(* Logix 5000 Rung export; software revision 16.04 *)

MODULES
   Local : vendor None type None code None
   MVI69E_AFC : vendor None type None code None
END_MODULES

TYPE AFCESiteAlarms :   // Indicates if a meter has any alarms
STRUCT
   Meter1 : BOOL;   // Meter in alarm
   Meter2 : BOOL;   // Meter in alarm
   Meter3 : BOOL;   // Meter in alarm
   Meter4 : BOOL;   // Meter in alarm
   Meter5 : BOOL;   // Meter in alarm
   Meter6 : BOOL;   // Meter in alarm
   Meter7 : BOOL;   // Meter in alarm
   Meter8 : BOOL;   // Meter in alarm
   Meter9 : BOOL;   // Meter in alarm
   Meter10 : BOOL;   // Meter in alarm
   Meter11 : BOOL;   // Meter in alarm
   Meter12 : BOOL;   // Meter in alarm
   Meter13 : BOOL;   // Meter in alarm
   Meter14 : BOOL;   // Meter in alarm
   Meter15 : BOOL;   // Meter in alarm
   Meter16 : BOOL;   // Meter in alarm
END_STRUCT
END_TYPE

TYPE AFCEFlag :   // Flags contains status information updated by ladder and also trigger bits for clock update
STRUCT
   AFCStopped : BOOL;   // Indicates that the module has sent a new input block to be processed by ladder - UPDATED BY LADDER
   AFCInputSequenceNum : INT;   // Meter number (0 -15) associated to blocks 1-16. Used to update "Profile" (meter type and product group.) UPDATED BY LADDER
END_STRUCT
END_TYPE

TYPE AFCEUtilBlockNonInterrupt :
STRUCT
   Now : BOOL;
   ModbusMasterCommand : BOOL;
   ModbusMasterResponse : BOOL;
   Archive : DINT;
   Prover : BOOL;
   PassThru : BOOL;
   Calibration : BOOL;
END_STRUCT
END_TYPE

TYPE AFCEMeterCalRequestActionType :
STRUCT
   ZeroShift : BOOL;   // Zero Shift
   SetZero : BOOL;   // Set Zero
   SetSpan : BOOL;   // Set Span
   SetMid1 : BOOL;   // Set Mid 1
   SetMid2 : BOOL;   // Set Mid 2
   SetMid3 : BOOL;   // Set Mid 3
END_STRUCT
END_TYPE

TYPE AFCEMeterLinearGas :   // Linear Gas Meter
STRUCT
   Control : AFCEMeterControl;   // Meter Control
   Status : AFCEMeterStatus;   // Meter Status
   ProcessVariables : AFCEMeterLinearGasProcess;   // Input process variables to be transferred to the module
   Analysis : AFCEMeterAnalysis;   // Molar Analysis data to be transferred to the module (only for gas products with online gas chromatograph applications)
   Alarm : AFCEMeterLinearGasAlarm;   // Meter Alarms
   Archive : AFCEMeterLinearGasArchive;   // Archive
   Profile : AFCEMeterProfile;   // Module profile (meter type/product group) transfered from the module
   Calibration : AFCEMeterLinearGasCal;   // Calibration
   BackPlaneReturn : AFCEMeterLinearGasBackPlaneReturn;
END_STRUCT
END_TYPE

TYPE AFCEProveConfigEnable :   // Prove controls at enable
STRUCT
   MeterNumber : INT;   // Meter number requested (1-16)
   AutoAcceptProve : BOOL;   // Auto-accept the prove
   AutoContinueProve : BOOL;   // Auto-continue the prove
END_STRUCT
END_TYPE

TYPE AFCEModbusGateway :   // Modbus Gateway
STRUCT
   Command : AFCEModbusGatewayCommand[10];   // Modbus gateway commands - contains setup and modbus data
END_STRUCT
END_TYPE

TYPE AFCEMeterCalRequestActionValue :
STRUCT
   ZeroShift : AFCEMeterCalRequestValue;   // Zero Shift
   SetZero : AFCEMeterCalRequestValue;   // Set Zero
   SetSpan : AFCEMeterCalRequestValue;   // Set Span
   SetMid1 : AFCEMeterCalRequestValue;   // Set Mid 1
   SetMid2 : AFCEMeterCalRequestValue;   // Set Mid 2
   SetMid3 : AFCEMeterCalRequestValue;   // Set Mid 3
END_STRUCT
END_TYPE

TYPE AFCEMeterAnalysisError :
STRUCT
   StreamOutOfRange : BOOL;   // Requested Stream Number Out of Range
   StreamNotConfigured : BOOL;   // Requested Stream Not Configured
END_STRUCT
END_TYPE

TYPE AFCEMeterLinearGasArchiveWrite :   // Write Archive
STRUCT
   Daily : BOOL;   // Set to 1 to write daily archive
   Hourly : BOOL;   // Set to 1 to write hourly archive
END_STRUCT
END_TYPE

TYPE AFCEMeterCalRequestValue :
STRUCT
   Applied : REAL;   // Applied
   Measured : REAL;   // Measured
END_STRUCT
END_TYPE

TYPE AFCEModbusMasterDataType :   // Modbus master data type
STRUCT
   Bit : BOOL;   // bit type
   Word : BOOL;   // word type (16-bit)
   Long : BOOL;   // long integer (32-bit)
   LongRemote : BOOL;   // long integer (32-bit)
END_STRUCT
END_TYPE

TYPE AFCEUtil :   // Used for internal ladder logic usage. These values must not be changed by user application.
STRUCT
   Flags : AFCEFlag;   // Wallclock update commands
   CycleCounter : INT;   // Reflects current block ID calculated by ladder to be sent to the module
   Buffer : AFCEUtilBuffer;
   Block : AFCEUtilBlock;
END_STRUCT
END_TYPE

TYPE AFCEWallclock :
STRUCT
   GetAFCTime : BOOL;   // Get current AFC Time
   SetAFCTimeFromPLCTime : BOOL;   // Set AFC time from PLC time. Updates current AFC time
   EnableLocalDateTime : BOOL;   // Enable Local Date Time.
   AFCTime : AFCETime;   // Coordinated Universal Time. Updated by either getting or setting AFC time.
END_STRUCT
END_TYPE

TYPE AFCEProvePhaseBitmap :   // AFC prove phase bitmap
STRUCT
   NotSelected : BOOL;   // Not selected
   Active : BOOL;   // Active, not counting
   CountingPast1stSwitch : BOOL;   // Counting past 1st switch for Udir and forward leg for Bdir)
   Past2ndSwitchFwdLeg : BOOL;   // Past 2nd switch forward leg (bidirectional only)
   Past1stSwithRetLeg : BOOL;   // Past 1st switch return leg (bidirectional only)
   RunComplete : BOOL;   // Run complete. past 2nd switch.
END_STRUCT
END_TYPE

TYPE AFCEMeterLinearGasCalRequest :
STRUCT
   ProcessVariable : AFCEMeterLinearGasCalRequestProces;   // Process Variable
   ActionType : AFCEMeterCalRequestActionType;   // Action Type
   Value : AFCEMeterCalRequestActionValue;   // Value
   Count : DINT;   // Number of calibration requests
END_STRUCT
END_TYPE

TYPE AFCEProveInputConfig :   // Prove input block results - prover configuration
STRUCT
   Type : INT;   // Prover type
   Options : INT;   // Prover options
   RunsPerProveTotal : INT;   // Total runs per prove
   RunsPerProveSelected : INT;   // Selected runs per prove
   MaxRunsBeforeAbort : INT;   // Max total runs before abort
   ShortPassesPerRun : INT;   // Short passes per run if bidir = 2 , else 0
END_STRUCT
END_TYPE

TYPE AFCEMeterCalResponse :
STRUCT
   Trigger : BOOL;   // Send Error Code and Values to module to be recorded
   ErrorCode : SINT;   // Error Code to send. 0-4 allowed. 0=No error. 1-4=User defined.
   Value : AFCEMeterCalRequestValue;   // Value to Send
   Count : DINT;   // Number of calibration responses
END_STRUCT
END_TYPE

TYPE AFCEMeterLinearGasAlarmControl :   // Linear Gas Process Alarms
STRUCT
   PulseFrequency : AFCEMeterProcessAlarm;   // Pulse Frequency Alarms
   Temperature : AFCEMeterProcessAlarm;   // Temperature Alarms
   Pressure : AFCEMeterProcessAlarm;   // Pressure Alarms
   MeterPulses : AFCEMeterProcessAlarmFidelity;   // Meter Pulses Alarms
END_STRUCT
END_TYPE

TYPE AFCEMeterArchiveFetchError :
STRUCT
   ArchiveSelectionInvalid : BOOL;   // Archive File Selection Invalid
   AgeOutsideSize : BOOL;   // Age Outside Configured File Size
   ArchiveNeverWritten : BOOL;   // Age OK but Archive Record Never Written (new or reconfigured meter)
   Reserverd1 : BOOL;
   Reserverd2 : BOOL;
   Reserverd3 : BOOL;
   Reserverd4 : BOOL;
   Reserverd5 : BOOL;
   Reserverd6 : BOOL;
   Reserverd7 : BOOL;
   Reserverd8 : BOOL;
   Reserverd9 : BOOL;
   Reserverd10 : BOOL;
   Reserverd11 : BOOL;
   Reserverd12 : BOOL;
   Reserverd13 : BOOL;
END_STRUCT
END_TYPE

TYPE AFCEModbusGatewayCommand :   // Modbus Gateway Command
STRUCT
   Config : AFCEModbusGatewayConfig;   // Config data to be entered by the user.
   Trigger : BOOL;   // Trigger the Command, when cleared module has responded.
   Data : INT[200];   // Contains modbus data written to the module (write commands)
END_STRUCT
END_TYPE

TYPE AFCEProveConfigAccept :   // Prove controls at accept. If auto-accept is selected must be available at enable
STRUCT
   RequestedInterpolationPoint : INT;   // Requested interpolation point (0 nearest)
   ApplyMFChangeAllStreams : BOOL;   // Apply change in meter factor to all streams
   ApplyMFChangeCurve : BOOL;   // Apply change in meter factor to all curve points
   ApplyNewMF : BOOL;   // CApply new meter factor
END_STRUCT
END_TYPE

TYPE AFCEModbusMasterCommand :   // Modbus Master Command
STRUCT
   Config : AFCEModbusMasterConfig;   // Modbus Master Configuration
   ErrorCode : INT;   // Error Code associated to Modbus Master Command
   Pending : BOOL;   // Pending Modbus Master Command - waiting for Modbus Response
   ReturnedTransactionID : DINT;   // Changes to Config.TransactionID value when response has returned.
   Data : INT[100];   // Read or Write Data
END_STRUCT
END_TYPE

TYPE AFCEMeterStatusMeter :   // Meter Status
STRUCT
   Enabled : BOOL;   // Meter Enable Status, 1=enabled
   EnableAlarm : BOOL;   // If set either: 1. The meter is not configured. 2. The event log is full, the action was not performed.
END_STRUCT
END_TYPE

TYPE AFCEMeterControl :   // Enable/Disable Meter and Streams
STRUCT
   Meter : AFCEMeterControlMeter;   // Control the Meter
   Stream : AFCEMeterControlStream;   // Control the Meter Streams
   ResetAccumulators : AFCEMeterSignals;   // Resets for meter accumulators
END_STRUCT
END_TYPE

TYPE AFCEProveSequencing :   // AFC prove sequencing tag for phase selection and ball positioning
STRUCT
   Phase : AFCEProvePhaseBitmap;   // AFC phase sequencing
   BallPositionReady : BOOL;   // Ball position: Ready (Udir & Bdir only; fwd leg Bdir)
   BallPositionSealed : BOOL;   // Ball position: Sealed (Udir & Bdir only; fwd leg Bdir)
   BallPositionReadyBwdLeg : BOOL;   // Ball position: Ready bwd leg (Bdir only)
   BallPositionSealedBwdLeg : BOOL;   // Ball position: Sealed bwd leg (Bdir only)
END_STRUCT
END_TYPE

TYPE AFCEMeterLinearGasAlarm :
STRUCT
   Control : AFCEMeterLinearGasAlarmControl;   // Alarm Control
END_STRUCT
END_TYPE

TYPE AFCEUtilBlockInterrupt :
STRUCT
   Now : BOOL;
   ModbusGateway : DINT;
   EnableDisable : BOOL;
   Analysis : DINT;
END_STRUCT
END_TYPE

TYPE AFCEComponents :   // High precision gas component analysis (only supported version 2.07.000)
STRUCT
   C1 : REAL;   // Methane
   N2 : REAL;   // Nitrogen
   CO2 : REAL;   // Carbon Dioxide
   C2 : REAL;   // Ethane
   C3 : REAL;   // Propane
   H20 : REAL;   // Water
   H2S : REAL;   // Hydrogen Sulphide
   H2 : REAL;   // Hydrogen
   CO : REAL;   // Carbon Monoxide
   O2 : REAL;   // Oxygen
   IC4 : REAL;   // Iso-butane
   NC4 : REAL;   // Normal Butane
   IC5 : REAL;   // Iso-pentane
   NC5 : REAL;   // Normal-pentane
   C6 : REAL;   // Hexane
   C7 : REAL;   // Heptane
   C8 : REAL;   // Octane
   C9 : REAL;   // Nonane
   C10 : REAL;   // Decane
   He : REAL;   // Helium
   Ar : REAL;   // Argon
   NeoC5 : REAL;   // Not Used
   UxUser1 : REAL;   // Not Used
   UyUser2 : REAL;   // Not Used
   UxUser3 : REAL;   // Not Used
   UyUser4 : REAL;   // Not Used
   UxUser5 : REAL;   // Not Used
   UyUser6 : REAL;   // Not Used
   UxUser7 : REAL;   // Not Used
   UyUser8 : REAL;   // Not Used
   UxUser9 : REAL;   // Not Used
   UyUser10 : REAL;   // Not Used
END_STRUCT
END_TYPE

TYPE AFCEMeterStatus :   // Status
STRUCT
   Meter : AFCEMeterStatusMeter;   // Meter Status
   Stream : AFCEMeterStatusStream;   // Stream Status
END_STRUCT
END_TYPE

TYPE AFCEUtilBlock :
STRUCT
   ProcessInput : INT;
   InterruptPending : AFCEUtilBlockInterrupt;
   InterruptComplete : AFCEUtilBlockInterrupt;
   NonInterruptPending : AFCEUtilBlockNonInterrupt;
   NonInterruptComplete : AFCEUtilBlockNonInterrupt;
END_STRUCT
END_TYPE

TYPE AFCEModbusGatewayConfig :   // Modbus Ggateway Configuration
STRUCT
   Enable : BOOL;   // Set to 1 to enable modbus gateway command (0=disable)
   StartRegister : DINT;   // Start modbus address
   RegisterCount : INT;   // Word count (200 max)
   FunctionType : BOOL;   // 0 = read command, 1 = write command
   RegisterType : BOOL;   // 0 = holding register, 1 = input register
   SlaveType : BOOL;   // 0 = primary slave, 1 = virtual slave
END_STRUCT
END_TYPE

TYPE AFCEMeterControlMeter :   // Enable and Disable Meter
STRUCT
   Enable : BOOL;   // Enable the Meter
   Disable : BOOL;   // Disable the Meter
END_STRUCT
END_TYPE

TYPE AFCEMeterProfile :   // Meter configuration profile
STRUCT
   MeterType : BOOL;   // 0=Differential, 1=Linear
   ProductGroup : BOOL;   // 0=Gas, 1=Liquid
   PrimaryInput : BOOL;   // For differential, 0=Differential Pressure 1=Flow Rate. For Linear, 0=Pulse Count 1=Pulse Frequency
   AOIMismatch : BOOL;   // AOI Meter type does not match module for meter number
END_STRUCT
END_TYPE

TYPE AFCEModbusPassThru :   // AFC Modbus Pass-thru
STRUCT
   Enable : BOOL;   // Set to 1 to enable pass-thru functionality (requires AFC Manager setting)
   MessagePresent : BOOL;   // Message present in the response block
   GetMessage : BOOL;   // Get the pass-thru message. When the bit is cleared the message has been transferred to the PLC.
   FunctionBitWrite : BOOL;   // Function bit write
   OverflowError : BOOL;   // Overflow error flag
   ModbusAddress : INT;   // Destination modbus address
   RegisterCount : INT;   // Number of elements associated to command
   ReadDataWord : INT[125];   // Contains received data for word commands
   ReadDataBit : AFCEModbusPassThruBitData;   // Contains received data for bit commands
END_STRUCT
END_TYPE

TYPE AFCEUtilBuffer :   // Buffer
STRUCT
   Input : INT[248];   // Input buffer contains the complete block to be copied from the module
   Output : INT[247];   // Output buffer contains data the complete block to be copied to the module
   Process : INT[180];
   ArchiveDay : INT[98];
   ArchiveHour : INT[98];
   Prove : INT[26];
   Analysis : INT[198];
   MeterEnableDisable : INT[4];
   StreamEnable : INT[36];
   StreamDisable : INT[36];
   StreamSelect : INT[24];
   MeterSignals : INT[24];
   Calibration : INT[36];
END_STRUCT
END_TYPE

TYPE AFCEProveStatus :   // Status of the prove (returned from the module to the processor)
STRUCT
   ProveAccepted : BOOL;   // Prove was accepted
   MeterFactorApplied : BOOL;   // Meter factor was applied
   MFAppliedToCurve : BOOL;   // Meter factor was applied to all points in the curve
   MFAppliedToStreams : BOOL;   // Meter factor was applied to all streams
   ProveRejectedByCommand : BOOL;   // Prove was rejected by command
   ProveRejectedNoRuns : BOOL;   // Prove was rejected - empty prove (no runs)
   ProveRejectedDivideBy0 : BOOL;   // Prove was rejected - divide by 0
   ProveEnabled : BOOL;   // Prove is enabled
   ProvingRunInProgress : BOOL;   // Proving run is in progress
   ProveRejectedAbort : BOOL;   // Prove rejected: abort
   ProvePaused : BOOL;   // Prove is paused
   RunCancelled : BOOL;   // Run Is cancelled
   RunTimedOut : BOOL;   // Run timed out
END_STRUCT
END_TYPE

TYPE AFCEMeterStatusStreamAlarm :   // Stream Alarms
STRUCT
   StreamOutOfRange : BOOL;   // Requested Stream Number Out of Range
   StreamNotConfigured : BOOL;   // Requested Stream not Configured
   StreamNotEnabled : BOOL;   // Requested Stream not Enabled
   EventLogFull : BOOL;   // Event Log Full, Action not Performed
END_STRUCT
END_TYPE

TYPE AFCEMeterLinearGasCal :   // Processor Mediated Calibration
STRUCT
   Request : AFCEMeterLinearGasCalRequest;   // Calibration Request from module
   Response : AFCEMeterCalResponse;   // Processor Response
END_STRUCT
END_TYPE

TYPE AFCEMeterLinearGasProcess :   // Linear Gas Process Variables
STRUCT
   PulseFrequency : REAL;   // Pulse Frequency (Hz)
   Temperature : REAL;   // Temperature
   Pressure : REAL;   // Pressure
   MeterPulses : DINT;   // Pulse count
END_STRUCT
END_TYPE

TYPE AFCEProveConfig :   // Controls (configuration settings) associated to the prover
STRUCT
   Enable : AFCEProveConfigEnable;   // Controls at enable
   Accept : AFCEProveConfigAccept;   // Controls at accept
END_STRUCT
END_TYPE

TYPE AFCESiteStatus :   // Site status bits - contains general information about the module - not meter specific
STRUCT
   AFCActive : BOOL;   // AFC active
   ChecksumAlarms : BOOL;   // Checkum alarm active
   Reserved2 : BOOL;
   Reserved3 : BOOL;
   PLCHalted : BOOL;   // PLC in program mode or missing
   CfgChanged : BOOL;   // Configuration changed
   Powerup : BOOL;   // Module powered up
   ColdStart : BOOL;   // Module performed cold start (BBRAM initialized)
   ModbusMasterPending : BOOL;   // Modbus Master Poll Pending
   ModbusMasterComplete : BOOL;   // Modbus Master Poll Complete
   ModbusPassThruPending : BOOL;   // Modbus Pass-thru Input Pending
   CalibrationRequest : BOOL;   // Calibration request from module
   ProverEnabled : BOOL;   // Prover Enabled
   Reserved13 : BOOL;
   Reserved14 : BOOL;
   Reserved15 : BOOL;
END_STRUCT
END_TYPE

TYPE AFCEModbusMaster :   // Modbus Master. Port 3 must be configured as modbus master through AFC Manager to use this feature.
STRUCT
   Enable : BOOL;   // Enable the modbus master funcionality
   CommandIndex : INT;   // Selects which command index will be executed
   Command : AFCEModbusMasterCommand[10];   // Each command contains a specific modbus request to be sent out of the port
END_STRUCT
END_TYPE

TYPE AFCEProveProcess :   // Prove process output from processor to the module
STRUCT
   Sequencing : AFCEProveSequencing;   // Prover sequencing
   Temperature : REAL;   // Temperature for Single Probe provers. And Inlet Temperature for Dual Probe Provers.
   OutletTemperature : REAL;   // Outlet Temperature for Provers with Dual Probes.
   SwitchBarTemperature : REAL;   // Switch bar temperature
   Pressure : REAL;   // Pressure for Single Probe provers. And Inlet Pressure for Dual Probe Provers.
   OutletPressure : REAL;   // Outlet Pressure for Provers with Dual Probes.
   ProverDensity : REAL;   // Prover density
END_STRUCT
END_TYPE

TYPE AFCEExtended :
STRUCT
   Trigger : BOOL;
   Data : AFCEExtendedData;
END_STRUCT
END_TYPE

TYPE AFCEMeterSignals :   // Meter trigger accumulator and archive resets
STRUCT
   ResetAccumulator1 : BOOL;   // Set to 1 to reset resettable accumulator 1
   ResetAccumulator2 : BOOL;   // Set to 1 to reset resettable accumulator 2
   ResetAccumulator3 : BOOL;   // Set to 1 to reset resettable accumulator 3
   ResetAccumulator4 : BOOL;   // Set to 1 to reset resettable accumulator 4
END_STRUCT
END_TYPE

TYPE AFCEMeterProcessAlarm :   // Process Alarms
STRUCT
   SetGeneralFail : BOOL;   // Set to indicate General Failure of the Transmitter
   StaleData : BOOL;   // Clear to Indicate new process input data
   SetLowThreshold : BOOL;   // Set to indicate Lower Range Limit Exceeded
   SetHighThreshold : BOOL;   // Set to indicate Upper Range Limit Exceeded
   SetAutoClearStaleData : BOOL;   // Set to automatically clear stale data
END_STRUCT
END_TYPE

TYPE AFCEMeterLinearGasArchive :   // Linear Gas Archive
STRUCT
   Write : AFCEMeterLinearGasArchiveWrite;
   Fetch : AFCEMeterLinearGasArchiveFetch;
END_STRUCT
END_TYPE

TYPE AFCETime :   // AFC time format used for wallclock update.
STRUCT
   Year : DINT;   // Year
   Month : DINT;   // Month
   Day : DINT;   // Day
   Hour : DINT;   // Hour
   Minute : DINT;   // Minute
   second : DINT;   // Seconds
END_STRUCT
END_TYPE

TYPE AFCEModbusMasterSwap :   // Modbus master swap words/ swap bytes
STRUCT
   SwapWords : BOOL;   // Swap words
   SwapBytes : BOOL;   // Swap bytes
END_STRUCT
END_TYPE

TYPE AFCEMeterControlStream :
STRUCT
   Selected : SINT;   // Stream to Enable or Disable and/or make active.
   EnableSelected : BOOL;   // Enable the Selected Stream
   DisableSelected : BOOL;   // Disable the Selected Stream
   SetSelectedToActive : BOOL;   // Set Selected to Active Stream
END_STRUCT
END_TYPE

TYPE AFCEProvePulseCount :   // Values to be supplied at the end of the pass/run
STRUCT
   Meter : DINT;   // Meter pulse count
   MasterMeter : DINT;   // Master meter pulse count
END_STRUCT
END_TYPE

TYPE AFCEMeterStatusStream :
STRUCT
   Active : INT;   // Current Active Stream
   Enabled : AFCEMeterStatusStreamEnabled;   // Enabled Streams
   Configured : AFCEMeterStatusStreamEnabled;   // Configured Streams
   EnableAlarm : AFCEMeterStatusStreamAlarm;   // Enable Alarms
END_STRUCT
END_TYPE

TYPE AFCEExtendedData :
STRUCT
   Raw : INT[64];
END_STRUCT
END_TYPE

TYPE AFCEModbusPassThruBitData :   // AFC Modbus Pass-thru Bit Data
STRUCT
   Data : BOOL[2016];   // Contains received data for bit commands
END_STRUCT
END_TYPE

TYPE AFCEMeterLinearGasArchiveFetch :
STRUCT
   Daily : AFCEMeterLinearGasArchiveFetchT;
   Hourly : AFCEMeterLinearGasArchiveFetchT;
END_STRUCT
END_TYPE

TYPE AFCEModbusMasterConfig :   // Modbus master command settings
STRUCT
   Enable : BOOL;   // Set to 1 to enable command (0=disable)
   FunctionType : BOOL;   // Set to 1 to select write command (0=read command)
   RegisterBank : BOOL;   // Set to 1 to select input register (0=holding register)
   DataType : AFCEModbusMasterDataType;   // Select data type format
   SwapOption : AFCEModbusMasterSwap;   // Select byte and word swap (1 = swap, 0 = no swap)
   TypeSwap : INT;   // This value is calculated by ladder logic and must not be modified by user
   SlaveAddress : INT;   // Modbus slave address of remote device
   ModbusAddress : INT;   // Modbus data address on remote slave
   ElementCount : INT;   // Number of data elements (125 words)
   TransactionID : INT;   // Transaction ID. This value is returned to the ReturnedTransaction ID when the response has been received.
END_STRUCT
END_TYPE

TYPE AFCEMeterProcessAlarmFidelity :   // Process Alarms
STRUCT
   SetGeneralFail : BOOL;   // Set to indicate General Failure of the Transmitter
   StaleData : BOOL;   // Clear to Indicate new process input data
   Reserved : BOOL;   // Reserved
   SetPulseFidelityAlarm : BOOL;   // Set to indicate Pulse Fidelity Alarm
   SetAutoClearStaleData : BOOL;   // Set to automatically clear stale data
END_STRUCT
END_TYPE

TYPE AFCEMeterLinearGasStandardDataDflt :   // EAFC Backplane Return Standard Data
STRUCT
   Meter_Alarms : DINT;   // Meter alarms
   NR_Acc_Net_Totalizer : DINT;   // Non-resettable accumulator, net, totalizer (m3)
   NR_Acc_Net_Residue : REAL;   // Non-resettable accumulator, net, residue (m3)
   FlowRate_Net : REAL;   // Flow rate, net (m3/h)
   FlowRate_Gross : REAL;   // Flow rate, gross / indicated (m3/h)
   Ifpv : REAL;   // AGA 8, Supercompressibility, Fpv
   Cprime : REAL;   // C-prime
END_STRUCT
END_TYPE

TYPE AFCEMeterLinearGasBackPlaneReturn :   // Linear Gas Meter
STRUCT
   StandardDefault : AFCEMeterLinearGasStandardDataDflt;
   StandardRaw : INT[14];
   Extended : AFCEExtended;
END_STRUCT
END_TYPE

TYPE AFCEMeterLinearGasCalRequestProces :
STRUCT
   PulseFrequency : BOOL;   // Pulse Frequency
   Temperature : BOOL;   // Temperature
   Pressure : BOOL;   // Pressure
END_STRUCT
END_TYPE

TYPE AFCEMeterLinearGasArchiveDflt :   // Default Configuration
STRUCT
   ClosingTimestamp : DINT;
   CumulativeActiveStreams : INT;
   CurrentActiveStream : SINT;
   MeterStatus : SINT;
   FlowingPeriod : DINT;
   PeriodDuration : DINT;
   AccumulatorTotalizer : DINT;
   AccumulatorResidue : REAL;
   MeterAlarms : DINT;
   PulseFrequency : REAL;
   Temperature : REAL;
   Pressure : REAL;
   RelativeDensity : REAL;
   ReferenceCompressibility : REAL;
   FlowingCompressibility : REAL;
   Fpv : REAL;
   KFactor : REAL;
   MeterFactor : REAL;
   InputPulseCount : DINT;
   CurrentManPulseCount : DINT;
   MassNRAccumulatorCurrent : REAL;   // Non-resettable
   MassNRAccumulatorOpening : REAL;   // Non-resettable
   EnergyNRAccumulatorCurrent : REAL;   // Non-resettable
   EnergyNRAccumulatorOpening : REAL;   // Non-resettable
   NetNRAccumulatorCurrent : REAL;   // Non-resettable
   NetNRAccumulatorOpening : REAL;   // Non-resettable
   GrossNRAccumulatorCurrent : REAL;   // Non-resettable
   GrossNRAccumulatorOpening : REAL;   // Non-resettable
   MolarFractionComponent01_C1 : REAL;
   MolarFractionComponent02_N2 : REAL;
   MolarFractionComponent03_CO2 : REAL;
   MolarFractionComponent04_C2 : REAL;
   MolarFractionComponent05_C3 : REAL;
   MolarFractionComponent06_H2O : REAL;
   MolarFractionComponent07_H2S : REAL;
   MolarFractionComponent08_H2 : REAL;
   MolarFractionComponent09_CO : REAL;
   MolarFractionComponent10_O2 : REAL;
   MolarFractionComponent11_IC4 : REAL;
   MolarFractionComponent12_NC4 : REAL;
   MolarFractionComponent13_IC5 : REAL;
   MolarFractionComponent14_NC5 : REAL;
   MolarFractionComponent15_C6 : REAL;
   MolarFractionComponent16_C7 : REAL;
   MolarFractionComponent17_C8 : REAL;
   MolarFractionComponent18_C9 : REAL;
   MolarFractionComponent19_C10 : REAL;
   MolarFractionComponent20_He : REAL;
   MolarFractionComponent21_Ar : REAL;
   UserSpecifiedFlowAverage1 : REAL;
   UserSpecifiedFlowAverage2 : REAL;
   UserSpecifiedFlowAverage3 : REAL;
END_STRUCT
END_TYPE

TYPE AFCEModuleDef :   // Main user defined data type
STRUCT
   ModbusGateway : AFCEModbusGateway;   // Reads and write data between processor and module modbus table
   ModbusMaster : AFCEModbusMaster;   // Setup modbus master commands to be sent to remote slaves (through Port 3)
   ModbusPassThru : AFCEModbusPassThru;   // Modbus pass-thru data
   SiteStatus : AFCESiteStatus;   // Site status
   MeterAlarms : AFCESiteAlarms;   // Meter Alarms
   Prove : AFCEProve;   // Prover
   Wallclock : AFCEWallclock;   // Set clock and get clock information
   Firmware : AFCEFirmwareVersion;   // Firmware information
   Util : AFCEUtil;   // Used by ladder logic
END_STRUCT
END_TYPE

TYPE AFCEMeterAnalysis :   // Meter analysis components. Allows the processor to update molar analysis for low precision and high precision streams.
STRUCT
   Trigger : BOOL;   // Set to 1 to Send Updated Component Data to the Module
   Stream : INT;   // Stream for Analysis. Select 0 for current active stream.
   Error : AFCEMeterAnalysisError;   // Analysis Error
   Components : AFCEComponents;   // High precision gas components (floating point per component). Only supported for firmware version 2.07.000 or later
END_STRUCT
END_TYPE

TYPE AFCEProveSignals :   // Contains the proving signals that will trigger specific tasks from the module
STRUCT
   EnableProve : BOOL;   // Enables the prove
   AcceptProve : BOOL;   // Accepts the prove
   RejectProve : BOOL;   // Reject the prove
   RunStart : BOOL;   // Starts the run
   RunComplete : BOOL;   // Flags that the run is complete
   RunCancel : BOOL;   // Cancels the run
   RunDelete : BOOL;   // Deletes the run
   PassComplete : BOOL;   // Flag that the pass is complete
   PauseProve : BOOL;   // Pauses the Proving Process
   AbortProve : BOOL;   // Aborts the prove
END_STRUCT
END_TYPE

TYPE AFCEFirmwareVersion :
STRUCT
   Major : SINT;   // Major Version number
   Minor : SINT;   // Minor Version number
   Revision : INT;   // Revision
END_STRUCT
END_TYPE

TYPE AFCEMeterLinearGasArchiveFetchT :   // Fetch Archive
STRUCT
   Trigger : BOOL;   // Trigger Archive Fetch
   Age : INT;   // 0 = Current Archive
   Error : AFCEMeterArchiveFetchError;   // Archive Fetch Error
   Default : AFCEMeterLinearGasArchiveDflt;   // Default Archive
   Raw : INT[100];   // Raw Archive
END_STRUCT
END_TYPE

TYPE AFCEProveRunResults :   // Run results of the prove. Copied from the module to the pocessor
STRUCT
   CountAttempted : INT;   // Run count attempted
   CountCompleted : INT;   // Run count completed
   CountSelected : INT;   // Run count selected
   RunsSelected : INT;   // Bit Mapped Runs selected for calculations from completed runs
   NewMeterFactor : REAL;   // New meter factor
   ChangeInMeterFactor : REAL;   // Change in meter factor
END_STRUCT
END_TYPE

TYPE AFCEMeterStatusStreamEnabled :   // Stream Status 1 = Enabled
STRUCT
   Stream1 : BOOL;
   Stream2 : BOOL;
   Stream3 : BOOL;
   Stream4 : BOOL;
   Stream5 : BOOL;
   Stream6 : BOOL;
   Stream7 : BOOL;
   Stream8 : BOOL;
   Stream9 : BOOL;
   Stream10 : BOOL;
   Stream11 : BOOL;
   Stream12 : BOOL;
   Stream13 : BOOL;
   Stream14 : BOOL;
   Stream15 : BOOL;
   Stream16 : BOOL;
END_STRUCT
END_TYPE

TYPE AFCEProve :   // Prove
STRUCT
   Process : AFCEProveProcess;   // Process Variables
   Signals : AFCEProveSignals;   // AFC Prove Signals (triggers the proving update)
   Config : AFCEProveConfig;   // AFC Prove Control (configuration settings)
   PulseCounts : AFCEProvePulseCount;   // Pulse counts to be updated at the end of the run/pass
   ConfigInput : AFCEProveInputConfig;   // AFC prover input configuration
   Status : AFCEProveStatus;   // AFC prover status
   ErrorCode : INT;   // Prove error code
   ProveControlsEcho : INT;   // AFC module Echos the state of the Prove Controls
   RequestedMeterEcho : INT;   // AFC module Echos the Meter number requested
   RequestedCurvePointEcho : INT;   // AFC module Echos the requested Curve Point
   RunResults : AFCEProveRunResults;   // Prove and run results
   ProveEnabled : BOOL;   // ON if prove is enabled. This flag is coped from inputbuffer[247]
END_STRUCT
END_TYPE

ADD_ON_INSTRUCTION AOI69EAFCMeterLinearGas   (* revision 1.5, vendor ProSoft Technology Inc., ExecutePrescan *)
// Add-On instruction for the MVI69E-AFC.
// Linear Gas Meter
// Revision note:
// Updated  BackplaneReturn Tag name from ProcessInputs to Standard
// and ComponentAnalysis to Extended.
// Help:
// Compatible with version 4.04 of MVI69E-AFC firmware or higher.
// v1.1: Comp Analysis Return fix
// v1.2: Addition of default process input backplane return data mapping.
// v1.3: Made correlation changes between the Module Archive Default UDTs and the AOI Archive Default UDTs.
// v1.4: Made changes to the Flow Rate Primary Input Block ID Insertion in Rung 8 (Removed +1),
// Modified ModbusGatewayConfig UDT StartRegister Tag Data Type from INT to DINT.
// v1.5: Updated Tags names AFCMeterXXYYYYYY.BackPlaneReturn.ProcessInputs to
// AFCMeterXXYYYYYY.BackPlaneReturn.Standard and
// AFCMeterXXYYYYYY.BackPlaneReturn.ComponentAnalysis
//  to AFCMeterXXYYYYYY.BackPlaneReturn.Extended.
VAR_IN_OUT
   ConnectionInput : INT[248]; {required}
   AFC : AFCEModuleDef; {required}
   AFCMeter : AFCEMeterLinearGas; {required}
END_VAR
VAR_INPUT
   MeterNumber : SINT; {required}   // Meter Number Set to a number between 1 and 12
END_VAR
VAR
   StreamSelectedShift : DINT;
   StreamSelectBuffer : INT;
   EnabledStatusBuffer : INT;
   StreamSelectBlockID : DINT;
   StreamNumberShift : DINT;
   StreamErrorBuffer : DINT;
   StreamEnableBlockID : DINT;
   StreamEnableBitPosition : DINT;
   StreamDisableBlockID : DINT;
   ProfileBuffer : SINT[2];
   ProcessInputBlockID : DINT;
   AnalysisGroupBitPosition : INT;
   AnalysisErrorBuffer : INT;
   ProcessAlarmShifter : DINT;
   ProcessAlarmBuffer : DINT;
   MeterSignaltBlockID : DINT;
   MeterNumberShift : DINT;
   MeterNumberBitPostition : DINT;
   Inputbuffer : INT[248];
   CalibrationMeterNumberBuffer : DINT;
   CalibrationMediationPending : BOOL;
   CalibrationInputScalingIndex : DINT;
   CalibrationHandleBuffer : DINT;
   ArchiveStream : DINT;
   ArchiveMeterStatusRaw : DINT;
   ArchiveMeterStatusActiveStream : DINT;
   ArchiveCompleteBitCheck : DINT;
   ArchiveBlockID : DINT;
   AnalysisGroupShift : DINT;
   AnalysisCompleteBitCheck : DINT;
   AnalysisBufferOffset : DINT;
   AnalysisBlockID : DINT;
   AFCStopped : BOOL;
   AFCInputDataAvailable : BOOL;
END_VAR

ROUTINE Logic   (* ladder *)
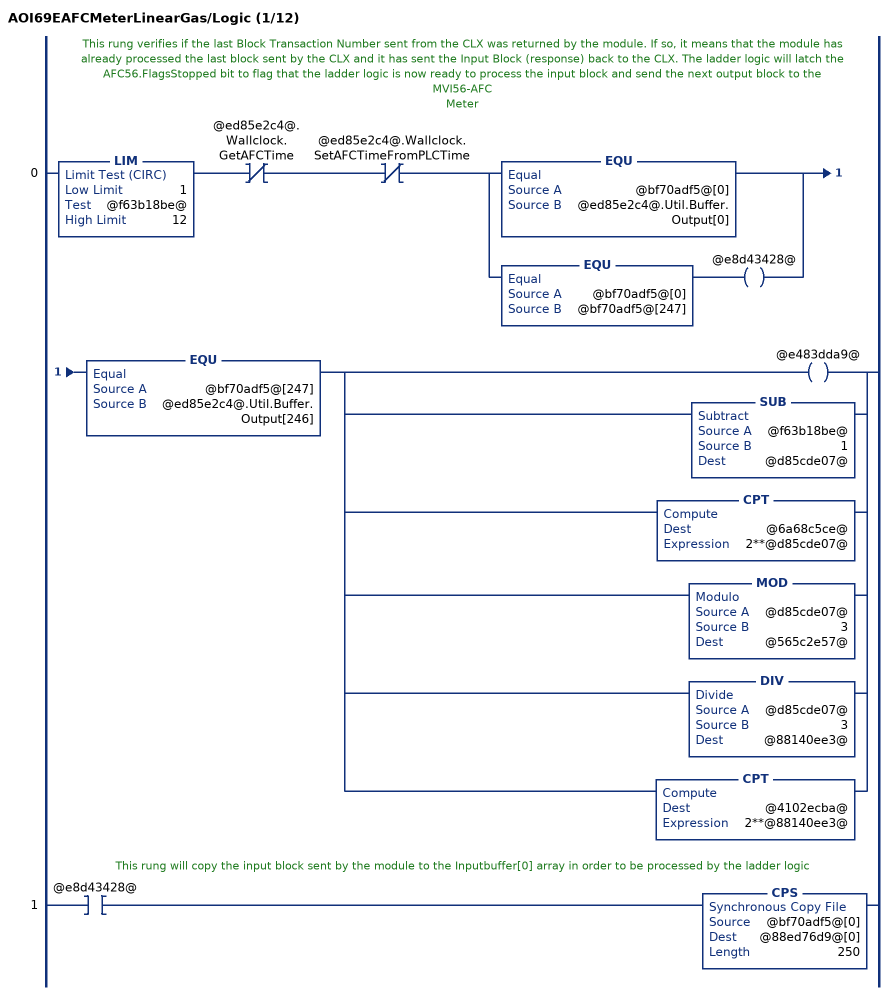
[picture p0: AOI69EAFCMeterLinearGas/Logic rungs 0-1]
   // This rung verifies if the last Block Transaction Number sent from the CLX was returned by the module. If so, it means that the module has already processed the last block sent by the CLX and it has sent the Input Block (response) back to the CLX. The ladder logic will latch the AFC56.FlagsStopped bit to flag that the ladder logic is now ready to process the input block and send the next output block to the MVI56-AFC
   // Meter
   0: LIM(1,@f63b18be@,12)XIO(@ed85e2c4@.Wallclock.GetAFCTime)XIO(@ed85e2c4@.Wallclock.SetAFCTimeFromPLCTime)[EQU(@bf70adf5@[0],@ed85e2c4@.Util.Buffer.Output[0]) ,EQU(@bf70adf5@[0],@bf70adf5@[247]) OTE(@e8d43428@) ]EQU(@bf70adf5@[247],@ed85e2c4@.Util.Buffer.Output[246])[OTE(@e483dda9@) ,SUB(@f63b18be@,1,@d85cde07@) ,CPT(@6a68c5ce@,2**@d85cde07@) ,MOD(@d85cde07@,3,@565c2e57@) ,DIV(@d85cde07@,3,@88140ee3@) ,CPT(@4102ecba@,2**@88140ee3@) ];
   // This rung will copy the input block sent by the module to the Inputbuffer[0] array in order to be processed by the ladder logic
   1: XIC(@e8d43428@)CPS(@bf70adf5@[0],@88ed76d9@[0],250);
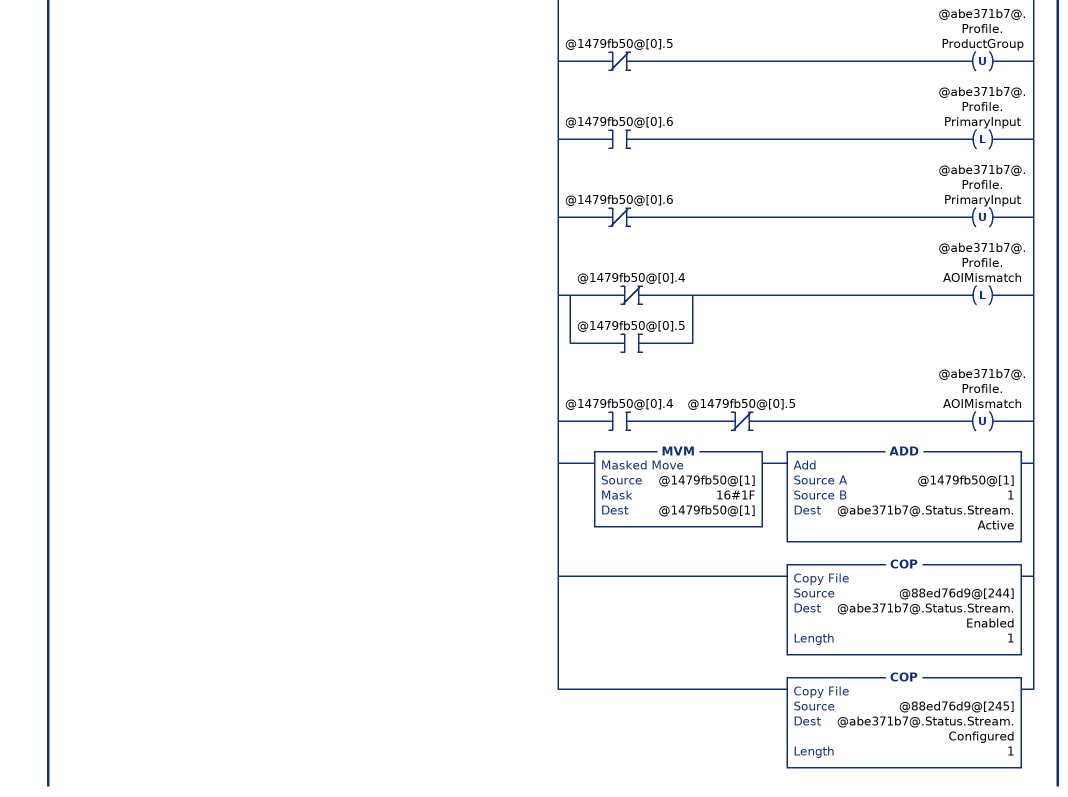
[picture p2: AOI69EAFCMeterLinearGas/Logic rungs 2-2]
   // Read process input backplane return and
   // meter profile (when block ID matches meter number).
   2: XIC(@e8d43428@)LIM(1,@88ed76d9@[0],12)[COP(@88ed76d9@[3+@d85cde07@*15],@abe371b7@.BackPlaneReturn.StandardRaw[0],14) ,COP(@abe371b7@.BackPlaneReturn.StandardRaw[0],@abe371b7@.BackPlaneReturn.StandardDefault,1) ,COP(@88ed76d9@[246],@ed85e2c4@.SiteStatus,1) ,EQU(@88ed76d9@[0],@f63b18be@) [COP(@88ed76d9@[243],@1479fb50@[0],2) ,[XIC(@1479fb50@[0].0) OTL(@abe371b7@.Status.Meter.EnableAlarm) ,XIO(@1479fb50@[0].0) OTU(@abe371b7@.Status.Meter.EnableAlarm) ] ,[XIC(@1479fb50@[0].1) OTL(@abe371b7@.Status.Meter.Enabled) ,XIO(@1479fb50@[0].1) OTU(@abe371b7@.Status.Meter.Enabled) ] ,[[XIC(@1479fb50@[0].4) OTL(@abe371b7@.Profile.MeterType) ,XIO(@1479fb50@[0].4) OTU(@abe371b7@.Profile.MeterType) ] ,[XIC(@1479fb50@[0].5) OTL(@abe371b7@.Profile.ProductGroup) ,XIO(@1479fb50@[0].5) OTU(@abe371b7@.Profile.ProductGroup) ] ,[XIC(@1479fb50@[0].6) OTL(@abe371b7@.Profile.PrimaryInput) ,XIO(@1479fb50@[0].6) OTU(@abe371b7@.Profile.PrimaryInput) ] ] ,[[XIO(@1479fb50@[0].4) ,XIC(@1479fb50@[0].5) ] OTL(@abe371b7@.Profile.AOIMismatch) ,XIC(@1479fb50@[0].4) XIO(@1479fb50@[0].5) OTU(@abe371b7@.Profile.AOIMismatch) ] ,MVM(@1479fb50@[1],16#1F,@1479fb50@[1]) ADD(@1479fb50@[1],1,@abe371b7@.Status.Stream.Active) ,COP(@88ed76d9@[244],@abe371b7@.Status.Stream.Enabled,1) ,COP(@88ed76d9@[245],@abe371b7@.Status.Stream.Configured,1) ] ];
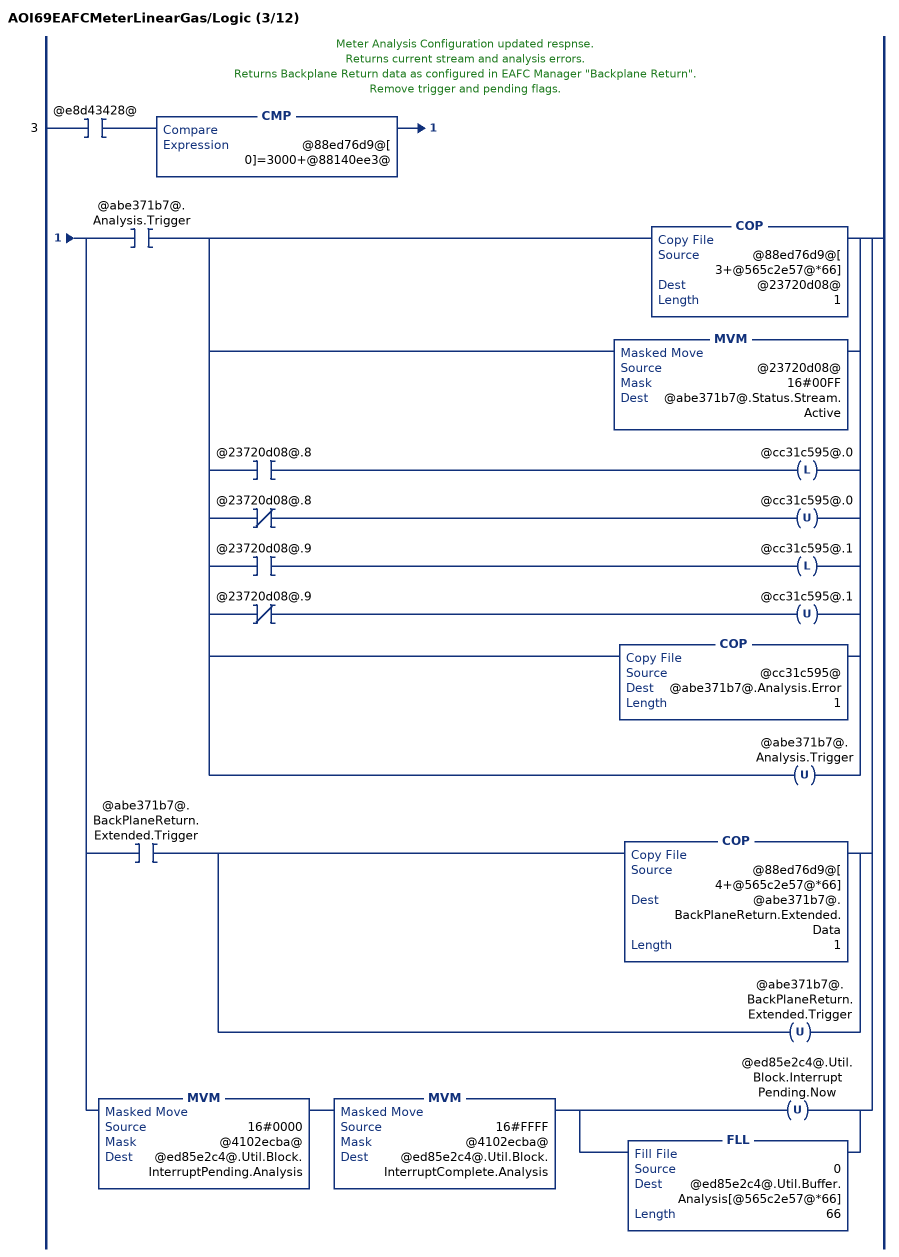
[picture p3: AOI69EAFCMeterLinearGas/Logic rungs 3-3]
   // Meter Analysis Configuration updated respnse.
   // Returns current stream and analysis errors.
   // Returns Backplane Return data as configured in EAFC Manager "Backplane Return".
   // Remove trigger and pending flags.
   3: XIC(@e8d43428@)CMP(@88ed76d9@[0]=3000+@88140ee3@)[XIC(@abe371b7@.Analysis.Trigger) [COP(@88ed76d9@[3+@565c2e57@*66],@23720d08@,1) ,MVM(@23720d08@,16#00FF,@abe371b7@.Status.Stream.Active) ,[XIC(@23720d08@.8) OTL(@cc31c595@.0) ,XIO(@23720d08@.8) OTU(@cc31c595@.0) ] ,[XIC(@23720d08@.9) OTL(@cc31c595@.1) ,XIO(@23720d08@.9) OTU(@cc31c595@.1) ] ,COP(@cc31c595@,@abe371b7@.Analysis.Error,1) ,OTU(@abe371b7@.Analysis.Trigger) ] ,XIC(@abe371b7@.BackPlaneReturn.Extended.Trigger) [COP(@88ed76d9@[4+@565c2e57@*66],@abe371b7@.BackPlaneReturn.Extended.Data,1) ,OTU(@abe371b7@.BackPlaneReturn.Extended.Trigger) ] ,MVM(16#0000,@4102ecba@,@ed85e2c4@.Util.Block.InterruptPending.Analysis) MVM(16#FFFF,@4102ecba@,@ed85e2c4@.Util.Block.InterruptComplete.Analysis) [OTU(@ed85e2c4@.Util.Block.InterruptPending.Now) ,FLL(0,@ed85e2c4@.Util.Buffer.Analysis[@565c2e57@*66],66) ] ];
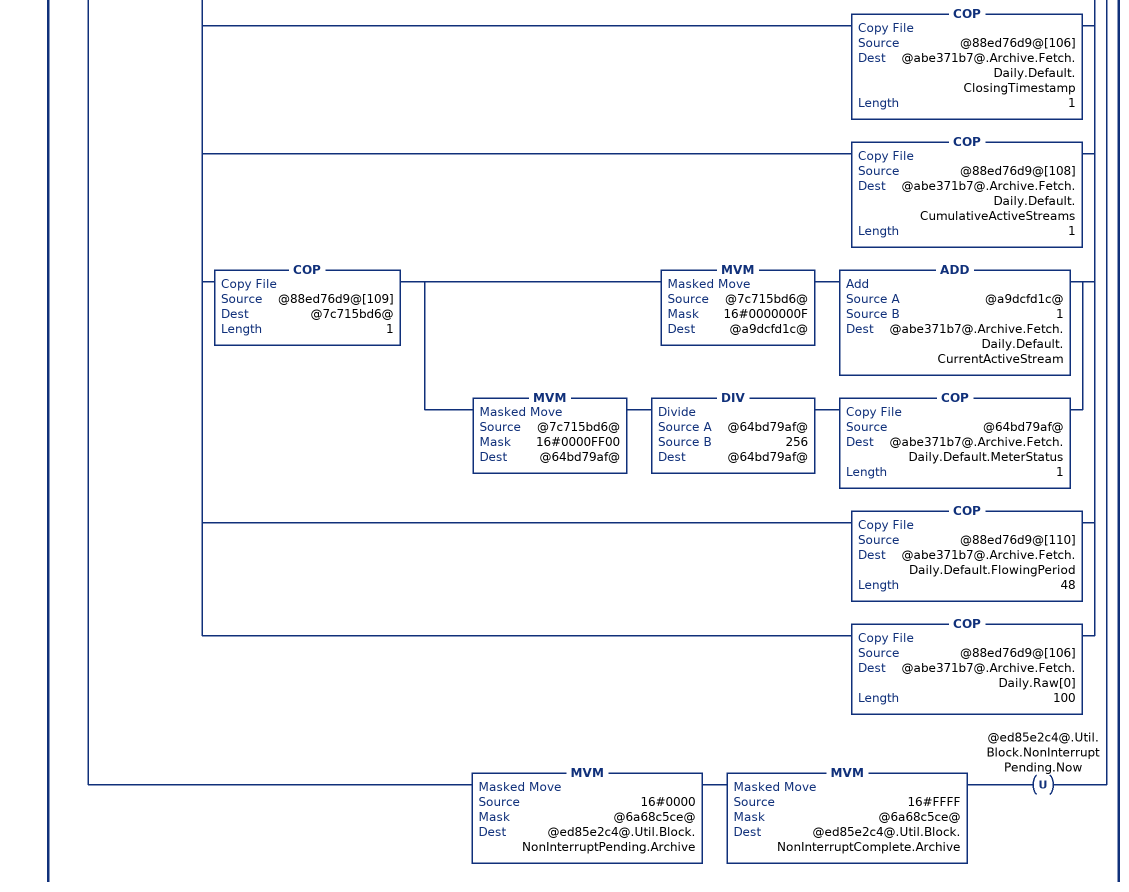
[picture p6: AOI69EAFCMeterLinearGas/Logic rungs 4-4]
   // Archive Fetch to default and raw UDT's.
   // Get archive alarms.
   // Remove trigger and pending flags.
   4: XIC(@e8d43428@)CMP(@88ed76d9@[0]=6000+@d85cde07@)[XIC(@abe371b7@.Archive.Fetch.Hourly.Trigger) [OTU(@abe371b7@.Archive.Fetch.Hourly.Trigger) ,[[XIC(@88ed76d9@[3].0) OTL(@abe371b7@.Archive.Fetch.Hourly.Error.ArchiveSelectionInvalid) ,XIO(@88ed76d9@[3].0) OTU(@abe371b7@.Archive.Fetch.Hourly.Error.ArchiveSelectionInvalid) ] ,[XIC(@88ed76d9@[3].1) OTL(@abe371b7@.Archive.Fetch.Hourly.Error.AgeOutsideSize) ,XIO(@88ed76d9@[3].1) OTU(@abe371b7@.Archive.Fetch.Hourly.Error.AgeOutsideSize) ] ,[XIC(@88ed76d9@[3].2) OTL(@abe371b7@.Archive.Fetch.Hourly.Error.ArchiveNeverWritten) ,XIO(@88ed76d9@[3].2) OTU(@abe371b7@.Archive.Fetch.Hourly.Error.ArchiveNeverWritten) ] ] ,COP(@88ed76d9@[4],@abe371b7@.Archive.Fetch.Hourly.Default.ClosingTimestamp,1) ,COP(@88ed76d9@[6],@abe371b7@.Archive.Fetch.Hourly.Default.CumulativeActiveStreams,1) ,COP(@88ed76d9@[7],@7c715bd6@,1) [MVM(@7c715bd6@,16#0000000F,@a9dcfd1c@) ADD(@a9dcfd1c@,1,@abe371b7@.Archive.Fetch.Hourly.Default.CurrentActiveStream) ,MVM(@7c715bd6@,16#0000FF00,@64bd79af@) DIV(@64bd79af@,256,@64bd79af@) COP(@64bd79af@,@abe371b7@.Archive.Fetch.Hourly.Default.MeterStatus,1) ] ,COP(@88ed76d9@[8],@abe371b7@.Archive.Fetch.Hourly.Default.FlowingPeriod,48) ,COP(@88ed76d9@[4],@abe371b7@.Archive.Fetch.Hourly.Raw[0],100) ] ,XIC(@abe371b7@.Archive.Fetch.Daily.Trigger) [OTU(@abe371b7@.Archive.Fetch.Daily.Trigger) ,[[XIC(@88ed76d9@[105].0) OTL(@abe371b7@.Archive.Fetch.Daily.Error.ArchiveSelectionInvalid) ,XIO(@88ed76d9@[105].0) OTU(@abe371b7@.Archive.Fetch.Daily.Error.ArchiveSelectionInvalid) ] ,[XIC(@88ed76d9@[105].1) OTL(@abe371b7@.Archive.Fetch.Daily.Error.AgeOutsideSize) ,XIO(@88ed76d9@[105].1) OTU(@abe371b7@.Archive.Fetch.Daily.Error.AgeOutsideSize) ] ,[XIC(@88ed76d9@[105].2) OTL(@abe371b7@.Archive.Fetch.Daily.Error.ArchiveNeverWritten) ,XIO(@88ed76d9@[105].2) OTU(@abe371b7@.Archive.Fetch.Daily.Error.ArchiveNeverWritten) ] ] ,COP(@88ed76d9@[106],@abe371b7@.Archive.Fetch.Daily.Default.ClosingTimestamp,1) ,COP(@88ed76d9@[108],@abe371b7@.Archive.Fetch.Daily.Default.CumulativeActiveStreams,1) ,COP(@88ed76d9@[109],@7c715bd6@,1) [MVM(@7c715bd6@,16#0000000F,@a9dcfd1c@) ADD(@a9dcfd1c@,1,@abe371b7@.Archive.Fetch.Daily.Default.CurrentActiveStream) ,MVM(@7c715bd6@,16#0000FF00,@64bd79af@) DIV(@64bd79af@,256,@64bd79af@) COP(@64bd79af@,@abe371b7@.Archive.Fetch.Daily.Default.MeterStatus,1) ] ,COP(@88ed76d9@[110],@abe371b7@.Archive.Fetch.Daily.Default.FlowingPeriod,48) ,COP(@88ed76d9@[106],@abe371b7@.Archive.Fetch.Daily.Raw[0],100) ] ,MVM(16#0000,@6a68c5ce@,@ed85e2c4@.Util.Block.NonInterruptPending.Archive) MVM(16#FFFF,@6a68c5ce@,@ed85e2c4@.Util.Block.NonInterruptComplete.Archive) OTU(@ed85e2c4@.Util.Block.NonInterruptPending.Now) ];
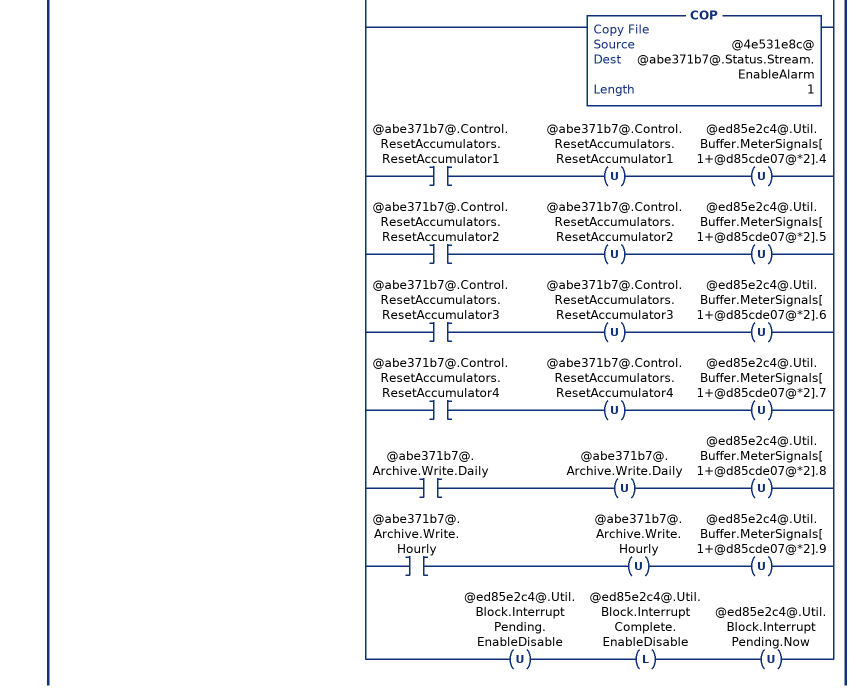
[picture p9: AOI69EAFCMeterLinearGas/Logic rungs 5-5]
   // Meter status and stream status.
   // Remove trigger and pending flags.
   5: XIC(@e8d43428@)EQU(@88ed76d9@[0],7000)[[MVM(@88ed76d9@[3],@6a68c5ce@,@da16ad6b@) ,[NEQ(@da16ad6b@,0) OTL(@abe371b7@.Status.Meter.Enabled) ,EQU(@da16ad6b@,0) OTU(@abe371b7@.Status.Meter.Enabled) ] ,OTU(@abe371b7@.Control.Meter.Enable) MVM(16#0000,@6a68c5ce@,@ed85e2c4@.Util.Buffer.MeterEnableDisable[1]) ,OTU(@abe371b7@.Control.Meter.Disable) MVM(16#0000,@6a68c5ce@,@ed85e2c4@.Util.Buffer.MeterEnableDisable[3]) ] ,[XIC(@abe371b7@.Control.Stream.EnableSelected) [COP(@88ed76d9@[7+@d85cde07@*3],@abe371b7@.Status.Stream.Enabled,1) ,COP(@88ed76d9@[8+@d85cde07@*3],@abe371b7@.Status.Stream.Configured,1) ,OTU(@abe371b7@.Control.Stream.EnableSelected) OTU(@abe371b7@.Control.Stream.DisableSelected) ] ,XIC(@abe371b7@.Control.Stream.DisableSelected) [COP(@88ed76d9@[55+@d85cde07@*3],@abe371b7@.Status.Stream.Enabled,1) ,COP(@88ed76d9@[56+@d85cde07@*3],@abe371b7@.Status.Stream.Configured,1) ,OTU(@abe371b7@.Control.Stream.EnableSelected) OTU(@abe371b7@.Control.Stream.DisableSelected) ] ] ,[OTU(@abe371b7@.Control.Stream.SetSelectedToActive) ,COP(@88ed76d9@[103+@d85cde07@*2],@23720d08@,1) ,[XIC(@23720d08@.8) OTL(@4e531e8c@.0) ,XIO(@23720d08@.8) OTU(@4e531e8c@.0) ] ,[XIC(@23720d08@.9) OTL(@4e531e8c@.1) ,XIO(@23720d08@.9) OTU(@4e531e8c@.1) ] ,[XIC(@23720d08@.10) OTL(@4e531e8c@.2) ,XIO(@23720d08@.10) OTU(@4e531e8c@.2) ] ,[XIC(@23720d08@.11) OTL(@4e531e8c@.3) ,XIO(@23720d08@.11) OTU(@4e531e8c@.3) ] ,MVM(@23720d08@,16#000F,@03251409@) ADD(@03251409@,1,@abe371b7@.Status.Stream.Active) ,COP(@4e531e8c@,@abe371b7@.Status.Stream.EnableAlarm,1) ] ,[XIC(@abe371b7@.Control.ResetAccumulators.ResetAccumulator1) OTU(@abe371b7@.Control.ResetAccumulators.ResetAccumulator1) OTU(@ed85e2c4@.Util.Buffer.MeterSignals[1+@d85cde07@*2].4) ,XIC(@abe371b7@.Control.ResetAccumulators.ResetAccumulator2) OTU(@abe371b7@.Control.ResetAccumulators.ResetAccumulator2) OTU(@ed85e2c4@.Util.Buffer.MeterSignals[1+@d85cde07@*2].5) ,XIC(@abe371b7@.Control.ResetAccumulators.ResetAccumulator3) OTU(@abe371b7@.Control.ResetAccumulators.ResetAccumulator3) OTU(@ed85e2c4@.Util.Buffer.MeterSignals[1+@d85cde07@*2].6) ,XIC(@abe371b7@.Control.ResetAccumulators.ResetAccumulator4) OTU(@abe371b7@.Control.ResetAccumulators.ResetAccumulator4) OTU(@ed85e2c4@.Util.Buffer.MeterSignals[1+@d85cde07@*2].7) ,XIC(@abe371b7@.Archive.Write.Daily) OTU(@abe371b7@.Archive.Write.Daily) OTU(@ed85e2c4@.Util.Buffer.MeterSignals[1+@d85cde07@*2].8) ,XIC(@abe371b7@.Archive.Write.Hourly) OTU(@abe371b7@.Archive.Write.Hourly) OTU(@ed85e2c4@.Util.Buffer.MeterSignals[1+@d85cde07@*2].9) ] ,OTU(@ed85e2c4@.Util.Block.InterruptPending.EnableDisable) OTL(@ed85e2c4@.Util.Block.InterruptComplete.EnableDisable) OTU(@ed85e2c4@.Util.Block.InterruptPending.Now) ];
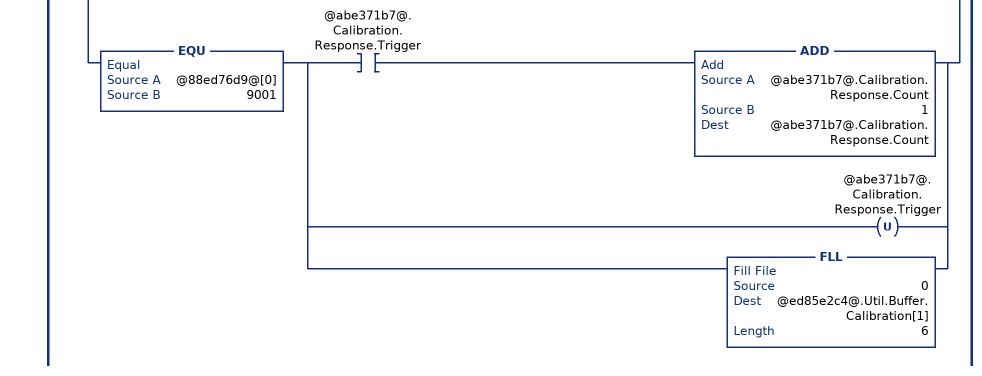
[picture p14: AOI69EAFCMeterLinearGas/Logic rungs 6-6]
   // Meter transmitter calibration.
   6: XIC(@e8d43428@)[EQU(@88ed76d9@[0],9000) ,EQU(@88ed76d9@[0],9001) ][MVM(@88ed76d9@[3],16#0F00,@624ee698@) ,DIV(@624ee698@,16#100,@624ee698@) ]EQU(@624ee698@,@d85cde07@)XIO(@88ed76d9@[3].14)[EQU(@88ed76d9@[0],9000) [XIO(@0ec75abb@) ADD(@abe371b7@.Calibration.Request.Count,1,@abe371b7@.Calibration.Request.Count) ,OTL(@0ec75abb@) [COP(@88ed76d9@[3],@6b8e262d@,1) ,MVM(@6b8e262d@,16#000F,@0e455032@) ] ,[EQU(@0e455032@,0) [OTL(@abe371b7@.Calibration.Request.ProcessVariable.PulseFrequency) ,OTU(@abe371b7@.Calibration.Request.ProcessVariable.Temperature) ,OTU(@abe371b7@.Calibration.Request.ProcessVariable.Pressure) ] ,EQU(@0e455032@,1) [OTL(@abe371b7@.Calibration.Request.ProcessVariable.Temperature) ,OTU(@abe371b7@.Calibration.Request.ProcessVariable.PulseFrequency) ,OTU(@abe371b7@.Calibration.Request.ProcessVariable.Pressure) ] ,EQU(@0e455032@,2) [OTL(@abe371b7@.Calibration.Request.ProcessVariable.Pressure) ,OTU(@abe371b7@.Calibration.Request.ProcessVariable.PulseFrequency) ,OTU(@abe371b7@.Calibration.Request.ProcessVariable.Temperature) ] ] ,[[XIC(@88ed76d9@[5].2) [OTL(@abe371b7@.Calibration.Request.ActionType.ZeroShift) ,COP(@88ed76d9@[6],@abe371b7@.Calibration.Request.Value.ZeroShift.Applied,2) ] ,XIO(@88ed76d9@[5].2) [OTU(@abe371b7@.Calibration.Request.ActionType.ZeroShift) ,FLL(0,@abe371b7@.Calibration.Request.Value.ZeroShift.Applied,2) ] ] ,[XIC(@88ed76d9@[5].3) [OTL(@abe371b7@.Calibration.Request.ActionType.SetZero) ,COP(@88ed76d9@[10],@abe371b7@.Calibration.Request.Value.SetZero.Applied,2) ] ,XIO(@88ed76d9@[5].3) [OTU(@abe371b7@.Calibration.Request.ActionType.SetZero) ,FLL(0,@abe371b7@.Calibration.Request.Value.SetZero.Applied,2) ] ] ,[XIC(@88ed76d9@[5].4) [OTL(@abe371b7@.Calibration.Request.ActionType.SetSpan) ,COP(@88ed76d9@[14],@abe371b7@.Calibration.Request.Value.SetSpan.Applied,2) ] ,XIO(@88ed76d9@[5].4) [OTU(@abe371b7@.Calibration.Request.ActionType.SetSpan) ,FLL(0,@abe371b7@.Calibration.Request.Value.SetSpan.Applied,2) ] ] ,[XIC(@88ed76d9@[5].5) [OTL(@abe371b7@.Calibration.Request.ActionType.SetMid1) ,COP(@88ed76d9@[18],@abe371b7@.Calibration.Request.Value.SetMid1.Applied,2) ] ,XIO(@88ed76d9@[5].5) [OTU(@abe371b7@.Calibration.Request.ActionType.SetMid1) ,FLL(0,@abe371b7@.Calibration.Request.Value.SetMid1.Applied,2) ] ] ,[XIC(@88ed76d9@[5].6) [OTL(@abe371b7@.Calibration.Request.ActionType.SetMid2) ,COP(@88ed76d9@[22],@abe371b7@.Calibration.Request.Value.SetMid2.Applied,2) ] ,XIO(@88ed76d9@[5].6) [OTU(@abe371b7@.Calibration.Request.ActionType.SetMid2) ,FLL(0,@abe371b7@.Calibration.Request.Value.SetMid2.Applied,2) ] ] ,[XIC(@88ed76d9@[5].7) [OTL(@abe371b7@.Calibration.Request.ActionType.SetMid3) ,COP(@88ed76d9@[26],@abe371b7@.Calibration.Request.Value.SetMid3.Applied,2) ] ,XIO(@88ed76d9@[5].7) [OTU(@abe371b7@.Calibration.Request.ActionType.SetMid3) ,FLL(0,@abe371b7@.Calibration.Request.Value.SetMid3.Applied,2) ] ] ] ] ,EQU(@88ed76d9@[0],9001) [XIC(@abe371b7@.Calibration.Response.Trigger) ADD(@abe371b7@.Calibration.Response.Count,1,@abe371b7@.Calibration.Response.Count) ,OTU(@abe371b7@.Calibration.Response.Trigger) ,FLL(0,@ed85e2c4@.Util.Buffer.Calibration[1],6) ] ];
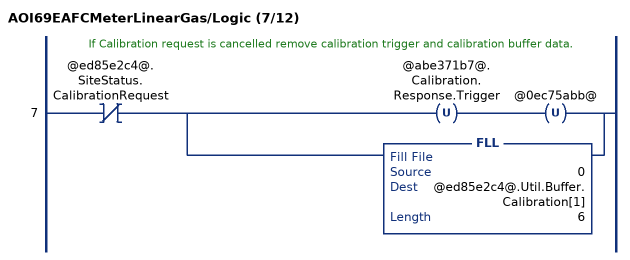
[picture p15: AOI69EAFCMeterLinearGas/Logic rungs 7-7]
   // If Calibration request is cancelled remove calibration trigger and calibration buffer data.
   7: XIO(@ed85e2c4@.SiteStatus.CalibrationRequest)[OTU(@abe371b7@.Calibration.Response.Trigger) OTU(@0ec75abb@) ,FLL(0,@ed85e2c4@.Util.Buffer.Calibration[1],6) ];
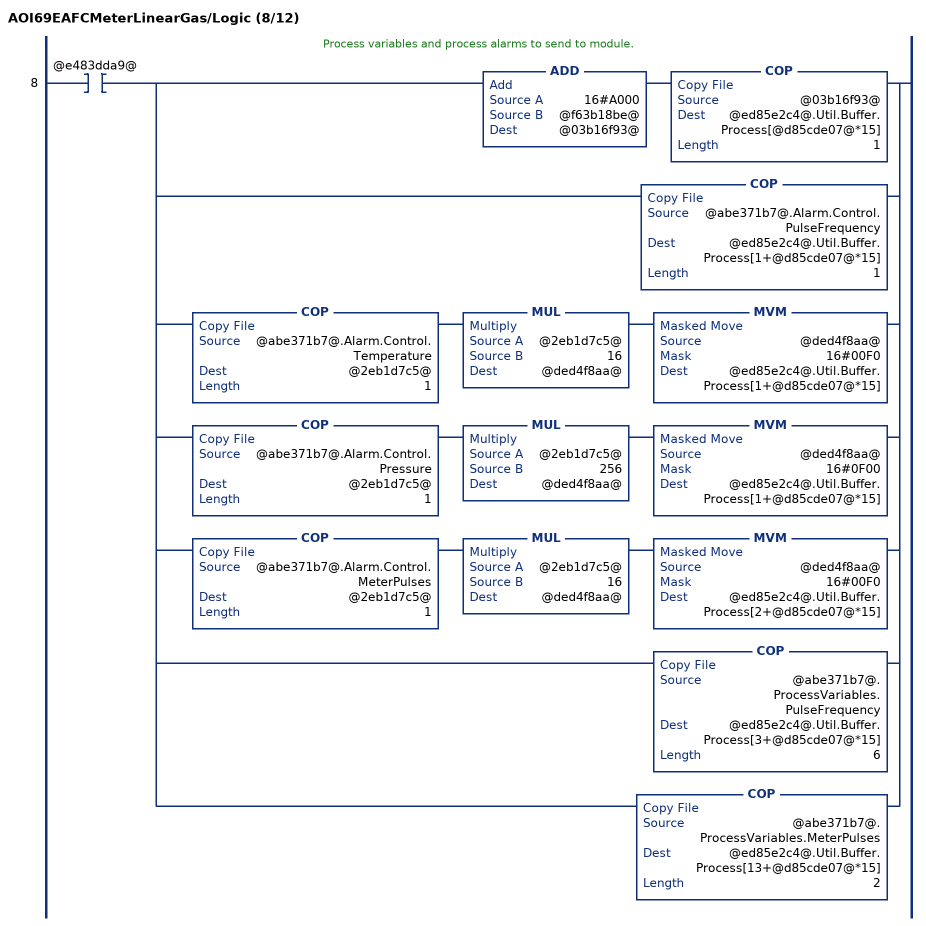
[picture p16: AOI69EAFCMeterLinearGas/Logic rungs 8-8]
   // Process variables and process alarms to send to module.
   8: XIC(@e483dda9@)[ADD(16#A000,@f63b18be@,@03b16f93@) COP(@03b16f93@,@ed85e2c4@.Util.Buffer.Process[@d85cde07@*15],1) ,COP(@abe371b7@.Alarm.Control.PulseFrequency,@ed85e2c4@.Util.Buffer.Process[1+@d85cde07@*15],1) ,COP(@abe371b7@.Alarm.Control.Temperature,@2eb1d7c5@,1) MUL(@2eb1d7c5@,16,@ded4f8aa@) MVM(@ded4f8aa@,16#00F0,@ed85e2c4@.Util.Buffer.Process[1+@d85cde07@*15]) ,COP(@abe371b7@.Alarm.Control.Pressure,@2eb1d7c5@,1) MUL(@2eb1d7c5@,256,@ded4f8aa@) MVM(@ded4f8aa@,16#0F00,@ed85e2c4@.Util.Buffer.Process[1+@d85cde07@*15]) ,COP(@abe371b7@.Alarm.Control.MeterPulses,@2eb1d7c5@,1) MUL(@2eb1d7c5@,16,@ded4f8aa@) MVM(@ded4f8aa@,16#00F0,@ed85e2c4@.Util.Buffer.Process[2+@d85cde07@*15]) ,[COP(@abe371b7@.ProcessVariables.PulseFrequency,@ed85e2c4@.Util.Buffer.Process[3+@d85cde07@*15],6) ,COP(@abe371b7@.ProcessVariables.MeterPulses,@ed85e2c4@.Util.Buffer.Process[13+@d85cde07@*15],2) ] ];
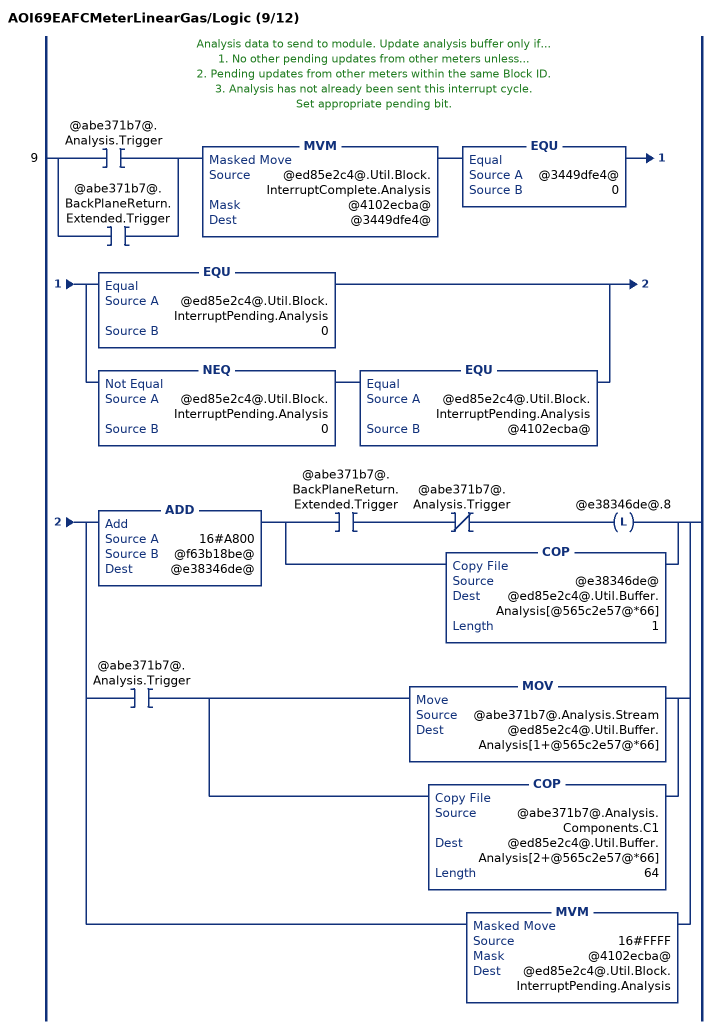
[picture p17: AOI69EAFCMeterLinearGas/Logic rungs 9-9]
   // Analysis data to send to module. Update analysis buffer only if...
   // 1. No other pending updates from other meters unless...
   // 2. Pending updates from other meters within the same Block ID.
   // 3. Analysis has not already been sent this interrupt cycle.
   // Set appropriate pending bit.
   9: [XIC(@abe371b7@.Analysis.Trigger) ,XIC(@abe371b7@.BackPlaneReturn.Extended.Trigger) ]MVM(@ed85e2c4@.Util.Block.InterruptComplete.Analysis,@4102ecba@,@3449dfe4@)EQU(@3449dfe4@,0)[EQU(@ed85e2c4@.Util.Block.InterruptPending.Analysis,0) ,NEQ(@ed85e2c4@.Util.Block.InterruptPending.Analysis,0) EQU(@ed85e2c4@.Util.Block.InterruptPending.Analysis,@4102ecba@) ][ADD(16#A800,@f63b18be@,@e38346de@) [XIC(@abe371b7@.BackPlaneReturn.Extended.Trigger) XIO(@abe371b7@.Analysis.Trigger) OTL(@e38346de@.8) ,COP(@e38346de@,@ed85e2c4@.Util.Buffer.Analysis[@565c2e57@*66],1) ] ,XIC(@abe371b7@.Analysis.Trigger) [MOV(@abe371b7@.Analysis.Stream,@ed85e2c4@.Util.Buffer.Analysis[1+@565c2e57@*66]) ,COP(@abe371b7@.Analysis.Components.C1,@ed85e2c4@.Util.Buffer.Analysis[2+@565c2e57@*66],64) ] ,MVM(16#FFFF,@4102ecba@,@ed85e2c4@.Util.Block.InterruptPending.Analysis) ];
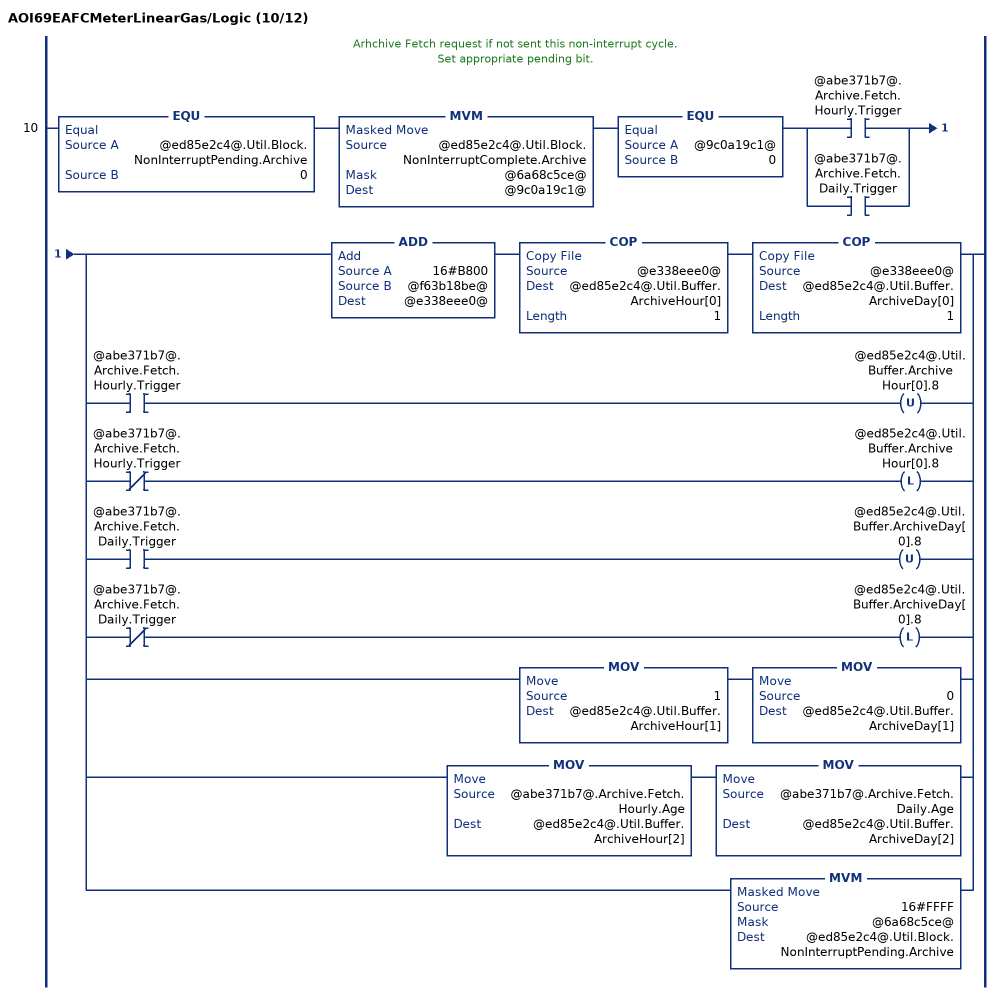
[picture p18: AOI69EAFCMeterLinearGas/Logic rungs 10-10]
   // Arhchive Fetch request if not sent this non-interrupt cycle.
   // Set appropriate pending bit.
   10: EQU(@ed85e2c4@.Util.Block.NonInterruptPending.Archive,0)MVM(@ed85e2c4@.Util.Block.NonInterruptComplete.Archive,@6a68c5ce@,@9c0a19c1@)EQU(@9c0a19c1@,0)[XIC(@abe371b7@.Archive.Fetch.Hourly.Trigger) ,XIC(@abe371b7@.Archive.Fetch.Daily.Trigger) ][ADD(16#B800,@f63b18be@,@e338eee0@) COP(@e338eee0@,@ed85e2c4@.Util.Buffer.ArchiveHour[0],1) COP(@e338eee0@,@ed85e2c4@.Util.Buffer.ArchiveDay[0],1) ,[XIC(@abe371b7@.Archive.Fetch.Hourly.Trigger) OTU(@ed85e2c4@.Util.Buffer.ArchiveHour[0].8) ,XIO(@abe371b7@.Archive.Fetch.Hourly.Trigger) OTL(@ed85e2c4@.Util.Buffer.ArchiveHour[0].8) ] ,[XIC(@abe371b7@.Archive.Fetch.Daily.Trigger) OTU(@ed85e2c4@.Util.Buffer.ArchiveDay[0].8) ,XIO(@abe371b7@.Archive.Fetch.Daily.Trigger) OTL(@ed85e2c4@.Util.Buffer.ArchiveDay[0].8) ] ,MOV(1,@ed85e2c4@.Util.Buffer.ArchiveHour[1]) MOV(0,@ed85e2c4@.Util.Buffer.ArchiveDay[1]) ,MOV(@abe371b7@.Archive.Fetch.Hourly.Age,@ed85e2c4@.Util.Buffer.ArchiveHour[2]) MOV(@abe371b7@.Archive.Fetch.Daily.Age,@ed85e2c4@.Util.Buffer.ArchiveDay[2]) ,MVM(16#FFFF,@6a68c5ce@,@ed85e2c4@.Util.Block.NonInterruptPending.Archive) ];
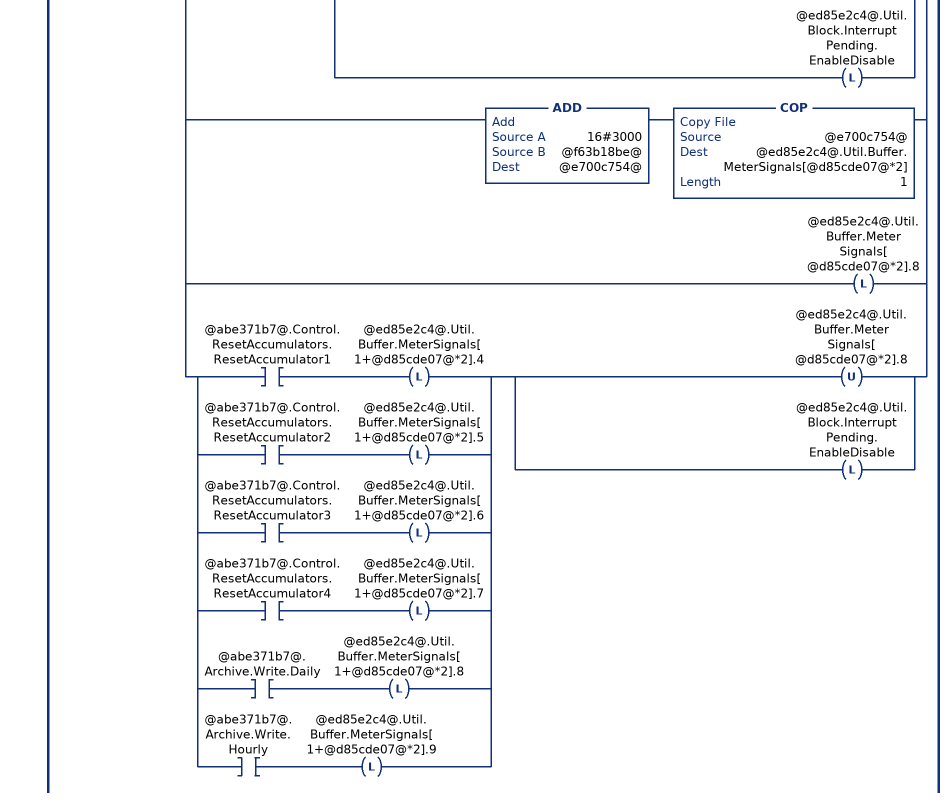
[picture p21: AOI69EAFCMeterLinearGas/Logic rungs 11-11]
   // Meter Enable.
   // Meter Disable.
   // Stream Select.
   // Stream Enable.
   // Stream Disable.
   // Set pending bit if not set this interrupt cycle.
   11: XIO(@ed85e2c4@.Util.Block.InterruptComplete.EnableDisable)[LIM(1,@abe371b7@.Control.Stream.Selected,16) CPT(@df6e64c6@,2**(@abe371b7@.Control.Stream.Selected-1)) ,[XIC(@abe371b7@.Control.Meter.Enable) MVM(16#FFFF,@6a68c5ce@,@ed85e2c4@.Util.Buffer.MeterEnableDisable[1]) MVM(16#0000,@6a68c5ce@,@ed85e2c4@.Util.Buffer.MeterEnableDisable[3]) ,XIC(@abe371b7@.Control.Meter.Disable) MVM(16#FFFF,@6a68c5ce@,@ed85e2c4@.Util.Buffer.MeterEnableDisable[3]) MVM(16#0000,@6a68c5ce@,@ed85e2c4@.Util.Buffer.MeterEnableDisable[1]) ] OTL(@ed85e2c4@.Util.Block.InterruptPending.EnableDisable) ,[ADD(16#CC00,@f63b18be@,@018cbb5f@) COP(@018cbb5f@,@ed85e2c4@.Util.Buffer.StreamEnable[@d85cde07@*3],1) ,XIO(@abe371b7@.Control.Stream.EnableSelected) OTL(@ed85e2c4@.Util.Buffer.StreamEnable[@d85cde07@*3].8) ,XIC(@abe371b7@.Control.Stream.EnableSelected) [OTU(@ed85e2c4@.Util.Buffer.StreamEnable[@d85cde07@*3].8) ,COP(@df6e64c6@,@ed85e2c4@.Util.Buffer.StreamEnable[1+@d85cde07@*3],1) ,OTL(@ed85e2c4@.Util.Block.InterruptPending.EnableDisable) ] ] ,[ADD(16#C800,@f63b18be@,@39ab54f1@) COP(@39ab54f1@,@ed85e2c4@.Util.Buffer.StreamDisable[@d85cde07@*3],1) ,XIO(@abe371b7@.Control.Stream.DisableSelected) OTL(@ed85e2c4@.Util.Buffer.StreamDisable[@d85cde07@*3].8) ,XIC(@abe371b7@.Control.Stream.DisableSelected) [OTU(@ed85e2c4@.Util.Buffer.StreamDisable[@d85cde07@*3].8) ,COP(@df6e64c6@,@ed85e2c4@.Util.Buffer.StreamDisable[1+@d85cde07@*3],1) ,OTL(@ed85e2c4@.Util.Block.InterruptPending.EnableDisable) ] ] ,[ADD(16#3C00,@f63b18be@,@3b20c622@) COP(@3b20c622@,@ed85e2c4@.Util.Buffer.StreamSelect[@d85cde07@*2],1) ,XIO(@abe371b7@.Control.Stream.SetSelectedToActive) OTL(@ed85e2c4@.Util.Buffer.StreamSelect[@d85cde07@*2].8) ,XIC(@abe371b7@.Control.Stream.SetSelectedToActive) [OTU(@ed85e2c4@.Util.Buffer.StreamSelect[@d85cde07@*2].8) ,MOV(@abe371b7@.Control.Stream.Selected,@ed85e2c4@.Util.Buffer.StreamSelect[1+@d85cde07@*2]) ,OTL(@ed85e2c4@.Util.Block.InterruptPending.EnableDisable) ] ] ,[ADD(16#3000,@f63b18be@,@e700c754@) COP(@e700c754@,@ed85e2c4@.Util.Buffer.MeterSignals[@d85cde07@*2],1) ,OTL(@ed85e2c4@.Util.Buffer.MeterSignals[@d85cde07@*2].8) ,[XIC(@abe371b7@.Control.ResetAccumulators.ResetAccumulator1) OTL(@ed85e2c4@.Util.Buffer.MeterSignals[1+@d85cde07@*2].4) ,XIC(@abe371b7@.Control.ResetAccumulators.ResetAccumulator2) OTL(@ed85e2c4@.Util.Buffer.MeterSignals[1+@d85cde07@*2].5) ,XIC(@abe371b7@.Control.ResetAccumulators.ResetAccumulator3) OTL(@ed85e2c4@.Util.Buffer.MeterSignals[1+@d85cde07@*2].6) ,XIC(@abe371b7@.Control.ResetAccumulators.ResetAccumulator4) OTL(@ed85e2c4@.Util.Buffer.MeterSignals[1+@d85cde07@*2].7) ,XIC(@abe371b7@.Archive.Write.Daily) OTL(@ed85e2c4@.Util.Buffer.MeterSignals[1+@d85cde07@*2].8) ,XIC(@abe371b7@.Archive.Write.Hourly) OTL(@ed85e2c4@.Util.Buffer.MeterSignals[1+@d85cde07@*2].9) ] [OTU(@ed85e2c4@.Util.Buffer.MeterSignals[@d85cde07@*2].8) ,OTL(@ed85e2c4@.Util.Block.InterruptPending.EnableDisable) ] ] ];
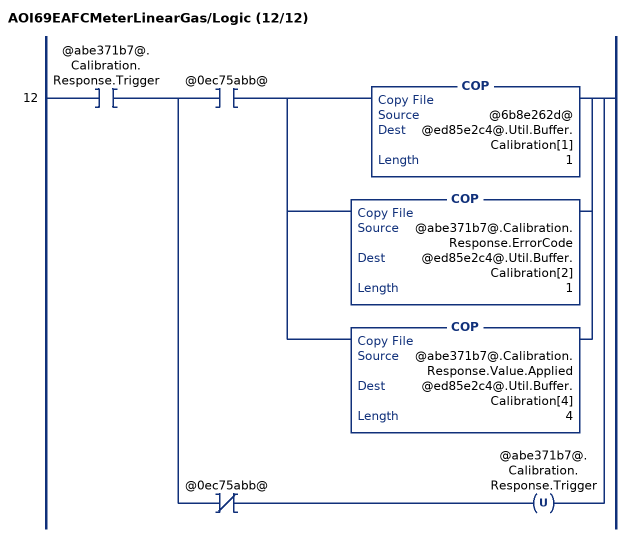
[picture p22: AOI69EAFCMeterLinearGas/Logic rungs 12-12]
   12: XIC(@abe371b7@.Calibration.Response.Trigger)[XIC(@0ec75abb@) [COP(@6b8e262d@,@ed85e2c4@.Util.Buffer.Calibration[1],1) ,COP(@abe371b7@.Calibration.Response.ErrorCode,@ed85e2c4@.Util.Buffer.Calibration[2],1) ,COP(@abe371b7@.Calibration.Response.Value.Applied,@ed85e2c4@.Util.Buffer.Calibration[4],4) ] ,XIO(@0ec75abb@) OTU(@abe371b7@.Calibration.Response.Trigger) ];
END_ROUTINE

ROUTINE Prescan   (* ladder *)
// Prescan
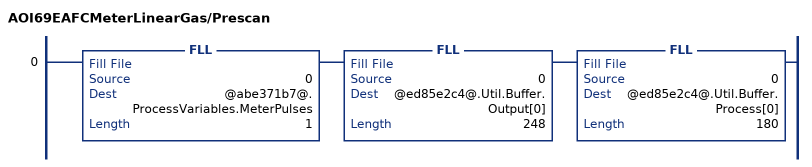
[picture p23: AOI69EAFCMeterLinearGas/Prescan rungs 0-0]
   0: FLL(0,@abe371b7@.ProcessVariables.MeterPulses,1)FLL(0,@ed85e2c4@.Util.Buffer.Output[0],248)FLL(0,@ed85e2c4@.Util.Buffer.Process[0],180);
END_ROUTINE
END_ADD_ON_INSTRUCTION

VAR_GLOBAL   (* controller tags *)
   AOI69EAFCMeter03LinearGas : AOI69EAFCMeterLinearGas;
   Local:1:I : AB:1756_MODULE_INT_496Bytes:I:0;
   AFC : AFCEModuleDef;
   AFCMeter03LinearGas : AFCEMeterLinearGas;
END_VAR

PROGRAM MainProgram

ROUTINE MainRoutine   (* ladder *)
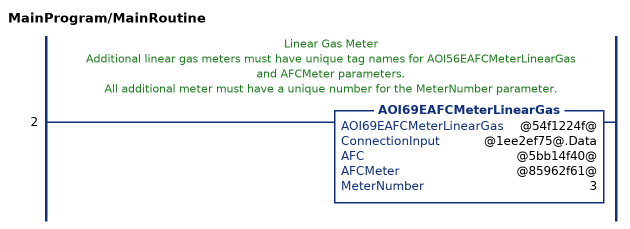
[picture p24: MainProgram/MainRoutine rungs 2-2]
   // Linear Gas Meter
   // Additional linear gas meters must have unique tag names for AOI56EAFCMeterLinearGas and AFCMeter parameters.
   // All additional meter must have a unique number for the MeterNumber parameter.
   2: AOI69EAFCMeterLinearGas(@54f1224f@,@1ee2ef75@.Data,@5bb14f40@,@85962f61@,3);
END_ROUTINE
END_PROGRAM
